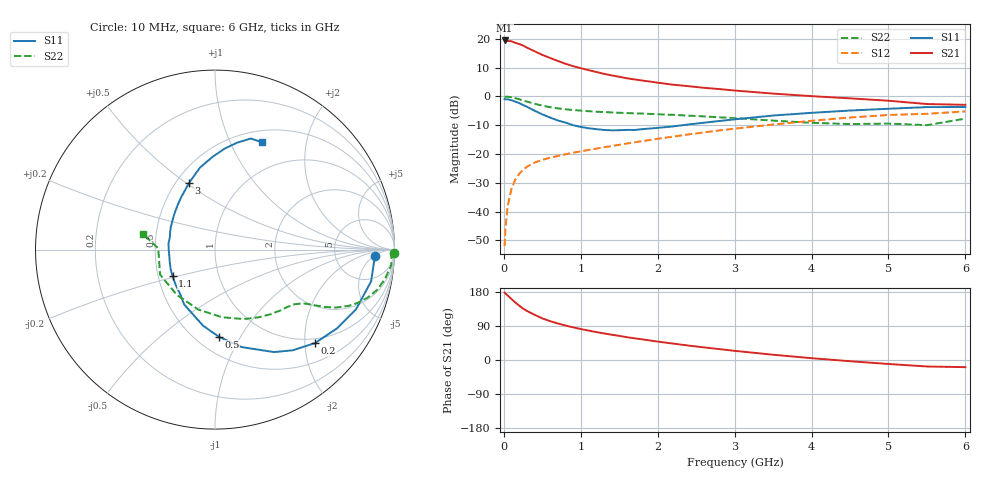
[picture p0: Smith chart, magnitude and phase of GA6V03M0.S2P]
! Infineon Technologies  Discrete & RF Semiconductors
! BF775
! Si NPN RF Bipolar Junction Transistor in SOT23
! VCE = 6 V  IC = 3 mA
! Common Emitter S-Parameters:  May  1996
# GHz  S  MA  R  50
!  f  S11  S21  S12  S22
! GHz  MAG  ANG  MAG  ANG  MAG  ANG  MAG  ANG
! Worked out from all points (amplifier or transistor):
!   36 points, 10 MHz to 6 GHz, reference 50 ohm
!   highest |S21| = 19.4 dB at 10 MHz (marker M1)
!   |S21| within 3 dB of that: start of sweep to 340.5 MHz
!   unconditionally stable (mu >= 1): 1.032 GHz to 3.257 GHz
!   at 250 MHz: K = 0.36, MSG = 21.6 dB, |S12| = -25.5 dB
!   at 1.4 GHz: K = 1.11, MAG = 10.3 dB, |S12| = -17.3 dB
!   at 6 GHz: K = 0.93, MSG = 1.1 dB, |S12| = -5.2 dB
!   S11 on the Smith chart (normalised r, x): 10 MHz: 16, -6; 200 MHz: 0.90, -2.23; 500 MHz: 0.64, -0.81; 1.1 GHz: 0.59, -0.19; 3 GHz: 0.58, +0.51; 6 GHz: 0.63, +1.32
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0.01  0.8948 -2.3  9.344 178.1  0.0025 93.2  0.9972 -1.0
0.02  0.8884 -4.7  9.181 175.8  0.0049 88.1  0.9833 -2.0
0.05  0.8877 -11.5  9.17 170.2  0.0125 83.7  0.9863 -5.0
0.1  0.8534 -22.9  9.034 160.9  0.0249 78.5  0.9613 -9.8
0.15  0.8089 -32.9  8.502 151.3  0.036 71.6  0.9294 -14.1
0.2  0.7632 -43.0  8.098 143.4  0.0451 67.1  0.891 -17.5
0.25  0.7083 -52.4  7.612 135.8  0.0532 63.2  0.8483 -20.5
0.3  0.6586 -60.1  7.019 129.5  0.0599 60.7  0.8086 -22.8
0.4  0.5626 -74.8  6.064 119.3  0.0707 56.0  0.7445 -25.7
0.5  0.486 -87.5  5.25 109.8  0.0789 53.5  0.6895 -27.6
0.6  0.4291 -98.9  4.647 102.6  0.0859 52.4  0.6479 -28.8
0.7  0.3815 -108.7  4.122 96.5  0.0921 51.8  0.6194 -29.8
0.9  0.3151 -128.0  3.345 86.2  0.105 51.5  0.579 -31.3
1.1  0.2791 -148.0  2.854 77.7  0.1171 52.3  0.5523 -33.2
1.3  0.261 -165.1  2.464 70.2  0.1304 53.0  0.5328 -35.1
1.6  0.2614 172.2  2.06 60.2  0.1516 53.6  0.512 -38.9
2.2  0.3006 139.0  1.593 43.3  0.1998 53.0  0.4773 -48.8
3  0.3987 111.3  1.262 24.2  0.2748 48.4  0.4186 -67.6
3.5  0.4643 100.4  1.116 13.9  0.3241 43.7  0.3789 -84.0
4.5  0.5669 84.3  0.923 -3.2  0.4286 31.8  0.33 -130.1
5.5  0.6505 72.1  0.735 -17.1  0.4973 16.0  0.3162 178.8
6  0.6527 66.6  0.713 -18.9  0.548 11.6  0.41 167.7
